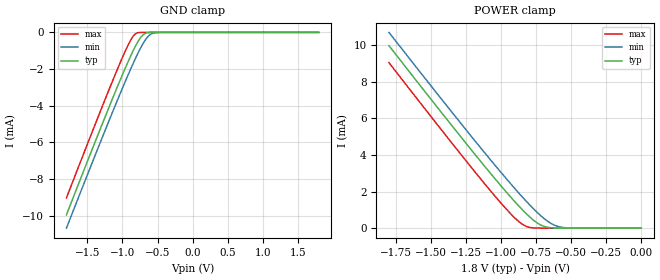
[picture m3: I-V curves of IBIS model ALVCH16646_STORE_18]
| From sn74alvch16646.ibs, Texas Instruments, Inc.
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[Model]   ALVCH16646_STORE_18
Model_type  Input
Vinl=0.5775
Vinh=1.2675
| variable   typ   min   max
C_comp   1.55pF   1.44pF   1.77pF
[Temperature Range]   40   100   -40
| Ambient temperature   25   85   -40
[Voltage range]   1.8   1.65   1.95
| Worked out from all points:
|   GND clamp passes 1 mA (typ) near -0.85 V on its own axis
|   POWER clamp passes 1 mA (typ) near -0.85 V on its own axis
[GND Clamp]
| ALVCH16646_STORE_18
|   Voltage   I(typ)   I(min)   I(max)
-1.8V     -9.965mA   -10.69mA   -9.037mA
-1.195V   -4.113mA   -4.852mA   -3.157mA
-1.02V    -2.488mA   -3.223mA   -1.541mA
-910mV    -1.517mA   -2.236mA   -620.7uA
-865mV    -1.143mA   -1.846mA   -310.6uA
-825mV    -828.8uA   -1.509mA   -114.4uA
-740mV    -277.1uA   -845.2uA   -3.141uA
-685mV    -77.5uA    -479.1uA   -219.8nA
-610mV    -6.621uA   -137.5uA   -5.748nA
-550mV    -770.8nA   -30.65uA   -316.1pA
-455mV    -24.82nA   -1.866uA   -8.05pA
1.8V      3.325pA    181.7pA    2.876pA
[POWER Clamp]
| ALVCH16646_STORE_18
|   Voltage   I(typ)   I(min)   I(max)
-1.8V     9.965mA    10.69mA    9.037mA
-1.38V    5.878mA    6.614mA    4.929mA
-1.105V   3.269mA    4.008mA    2.314mA
-940mV    1.776mA    2.501mA    856.4uA
-885mV    1.307mA    2.018mA    440uA
-845mV    982.9uA    1.676mA    200.1uA
-795mV    611.2uA    1.266mA    38.41uA
-715mV    166.7uA    670.1uA    941.7nA
-645mV    22.22uA    268.3uA    31.48nA
-585mV    2.717uA    77.14uA    1.709nA
-485mV    73.51nA    4.604uA    18.27pA
-16.28fV  3.324pA    5.122pA    3.398pA
